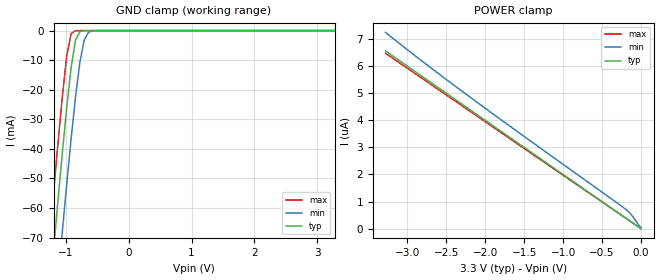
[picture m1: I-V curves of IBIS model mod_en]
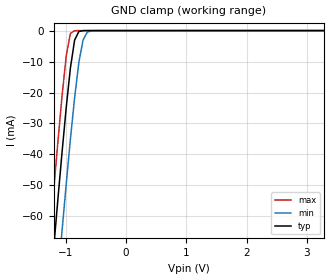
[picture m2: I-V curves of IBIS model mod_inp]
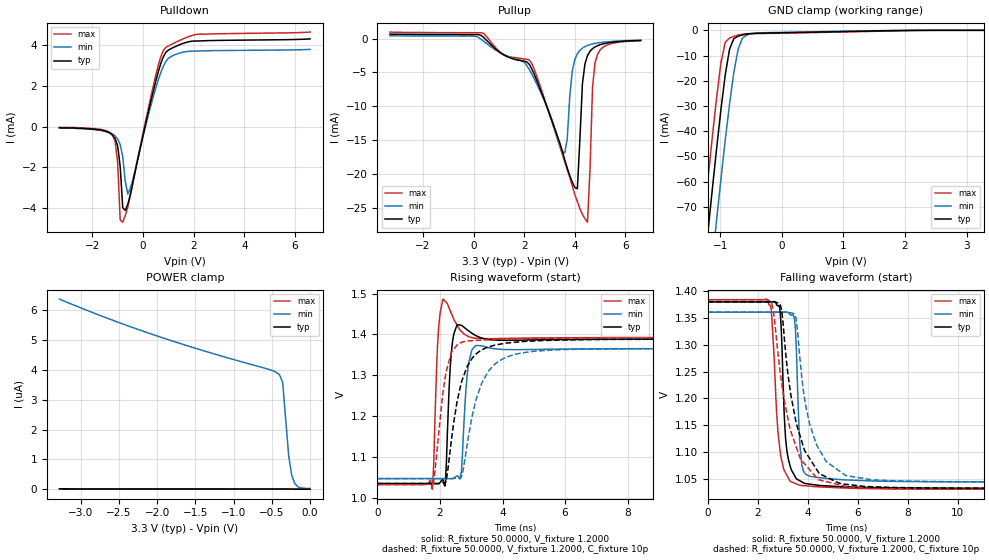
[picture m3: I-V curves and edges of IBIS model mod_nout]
| IBIS (I/O, Buffer, Information, Specification) Model, officially
| electronic behavioral standard for Buffer structures of digital pins.
[IBIS ver]  4.0
[File name] rhflvds2281.ibs
[File Rev]  1.0
[Date]   27 Jan 2015
[Source]   CAD & Design Services (Catania) - STMicroelectronics
[Notes]
   (Note1)  This IBIS model includes Ceramic Flat-64 package data
   (Note2)  This IBIS model has some Notes about the non-monotonicity
   of the I-V curves, but they are not indicative of problems
   inside the model;
[Copyright] (c) 2015 STMicroelectronics
|   Component RHFLVDS2281
[Component] RHFLVDS2281
[Manufacturer] STMicroelectronics
[Package]
| variable   typ   min   max
R_pkg   0.0   0.0   0.0
L_pkg   0.0H   0.0H   0.0H
C_pkg   0.0F   0.0F   0.0F
[Pin]  signal_name   model_name   R_pin   L_pin   C_pin
1   EN1   mod_en   NA   NA   NA
2   IN1P   mod_inp   NA   NA   NA
3   IN1N   mod_inn   NA   NA   NA
4   EN2   mod_en   NA   NA   NA
5   IN2P   mod_inp   NA   NA   NA
6   IN2N   mod_inn   NA   NA   NA
7   VCC   POWER   NA   NA   NA
8   GND   GND   NA   NA   NA
9   IN3P   mod_inp   NA   NA   NA
10   IN3N   mod_inn   NA   NA   NA
11   EN3   mod_en   NA   NA   NA
12   IN4P   mod_inp   NA   NA   NA
13   IN4N   mod_inn   NA   NA   NA
14   EN4   mod_en   NA   NA   NA
15   ENCK   mod_en   NA   NA   NA
16   CLKINP   mod_inp   NA   NA   NA
17   CLKINN   mod_inn   NA   NA   NA
18   GND   GND   NA   NA   NA
19   EN5   mod_en   NA   NA   NA
20   IN5P   mod_inp   NA   NA   NA
21   IN5N   mod_inn   NA   NA   NA
22   EN6   mod_en   NA   NA   NA
23   IN6P   mod_inp   NA   NA   NA
24   IN6N   mod_inn   NA   NA   NA
25   VCC   POWER   NA   NA   NA
26   GND   GND   NA   NA   NA
27   IN7P   mod_inp   NA   NA   NA
28   IN7N   mod_inn   NA   NA   NA
29   EN7   mod_en   NA   NA   NA
30   IN8P   mod_inp   NA   NA   NA
31   IN8N   mod_inn   NA   NA   NA
32   EN8   mod_en   NA   NA   NA
33   OUT8N   mod_nout   NA   NA   NA
34   OUT8P   mod_pout   NA   NA   NA
35   SL8   mod_sl   NA   NA   NA
36   OUT7N   mod_nout   NA   NA   NA
37   OUT7P   mod_pout   NA   NA   NA
38   SL7   mod_sl   NA   NA   NA
39   GND   GND   NA   NA   NA
40   VCC   POWER   NA   NA   NA
41   OUT6N   mod_nout   NA   NA   NA
42   OUT6P   mod_pout   NA   NA   NA
43   SL6   mod_sl   NA   NA   NA
44   OUT5N   mod_nout   NA   NA   NA
45   OUT5P   mod_pout   NA   NA   NA
46   SL5   mod_sl   NA   NA   NA
47   GND   GND   NA   NA   NA
48   CLKOUTN   mod_nout   NA   NA   NA
49   CLKOUTP   mod_pout   NA   NA   NA
50   VCC   POWER   NA   NA   NA
51   OUT4N   mod_nout   NA   NA   NA
52   OUT4P   mod_pout   NA   NA   NA
53   SL4   mod_sl   NA   NA   NA
54   OUT3N   mod_nout   NA   NA   NA
55   OUT3P   mod_pout   NA   NA   NA
56   SL3   mod_sl   NA   NA   NA
57   GND   GND   NA   NA   NA
58   VCC   POWER   NA   NA   NA
59   OUT2N   mod_nout   NA   NA   NA
60   OUT2P   mod_pout   NA   NA   NA
61   SL2   mod_sl   NA   NA   NA
62   OUT1N   mod_nout   NA   NA   NA
63   OUT1P   mod_pout   NA   NA   NA
64   SL1   mod_sl   NA   NA   NA
[Diff pin]  inv_pin   vdiff   tdelay_typ  tdelay_min  tdelay_max
2   3   200mV   0.0s   0.0s   0.0s
5   6   200mV   0.0s   0.0s   0.0s
9   10   200mV   0.0s   0.0s   0.0s
12   13   200mV   0.0s   0.0s   0.0s
16   17   200mV   0.0s   0.0s   0.0s
20   21   200mV   0.0s   0.0s   0.0s
23   24   200mV   0.0s   0.0s   0.0s
27   28   200mV   0.0s   0.0s   0.0s
30   31   200mV   0.0s   0.0s   0.0s
34   33   0.0V   0.0s   0.0s   0.0s
37   36   0.0V   0.0s   0.0s   0.0s
42   41   0.0V   0.0s   0.0s   0.0s
45   44   0.0V   0.0s   0.0s   0.0s
49   48   0.0V   0.0s   0.0s   0.0s
52   51   0.0V   0.0s   0.0s   0.0s
55   54   0.0V   0.0s   0.0s   0.0s
60   59   0.0V   0.0s   0.0s   0.0s
63   62   0.0V   0.0s   0.0s   0.0s
[Package Model]  302620_lvds2218
[Define Package Model]  302620_lvds2218
[Manufacturer]  STMicroelectronics
[OEM]  STMicroelectronics
[Description]  ceramic flat-64
[Number Of Pins]  64
[Pin Numbers]
|Pin Num   Terminal Name
1   | NET1:1
2   | NET2:2
3   | NET3:3
4   | NET4:4
5   | NET5:5
6   | NET6:6
7   | NET7:7
8   | NET8:8
9   | NET9:9
10   | NET10:10
11   | NET11:11
12   | NET12:12
13   | NET13:13
14   | NET14:14
15   | NET15:15
16   | NET16:16
17   | NET17:17
18   | NET18:18
19   | NET19:19
20   | NET20:20
21   | NET21:21
22   | NET22:22
23   | NET23:23
24   | NET24:24
25   | NET25:25
26   | NET26:26
27   | NET27:27
28   | NET28:28
29   | NET29:29
30   | NET30:30
31   | NET31:31
32   | NET32:32
33   | NET33:33
34   | NET34:34
35   | NET35:35
36   | NET36:36
37   | NET37:37
38   | NET38:38
39   | NET39:39
40   | NET40:40
41   | NET41:41
42   | NET42:42
43   | NET43:43
44   | NET44:44
45   | NET45:45
46   | NET46:46
47   | NET47:47
48   | NET48:48
49   | NET49:49
50   | NET50:50
51   | NET51:51
52   | NET52:52
53   | NET53:53
54   | NET54:54
55   | NET55:55
56   | NET56:56
57   | NET57:57
58   | NET58:58
59   | NET59:59
60   | NET60:60
61   | NET61:61
62   | NET62:62
63   | NET63:63
64   | NET64:64
[Model Data]
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[End Model Data]
[End Package Model]
| Models and submodels in the file (6): mod_en (Input), mod_inp (Input), mod_inn (Input), mod_nout (3-state), mod_pout (3-state), mod_sl (Input)
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|   Model mod_en
[Model]   mod_en
Model_type Input
Vinl   =   0.800V
Vinh   =   2.000V
C_comp   0.279pF   0.266pF   0.292pF
[Temperature Range]   25.0000   0.1250k   -55.0000
[Voltage Range]   3.3000V   3.0000V   3.6000V
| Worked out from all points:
|   GND clamp passes 1 mA (typ) near -0.80 V on its own axis
[GND_clamp]
|Voltage   I(typ)   I(min)   I(max)
-3.3V     -613.2mA   -637.8mA   -596mA
-1.27V    -91.5mA    -118.4mA   -72.02mA
-1.2V     -74.44mA   -101.4mA   -54.92mA
-1.13V    -57.71mA   -84.56mA   -38.25mA
-1.06V    -41.47mA   -68.06mA   -22.43mA
-990mV    -26.12mA   -52.01mA   -8.665mA
-920mV    -12.56mA   -36.67mA   -982.1uA
-850mV    -3.212mA   -22.55mA   -34.54uA
-780mV    -311.8uA   -10.71mA   -9.192uA
-710mV    -27.04uA   -3.134mA   -8.517uA
-570mV    -7.806uA   -73.26uA   -8.229uA
3.28V     -39.94nA   895.4nA    -631.5nA
[POWER_clamp]
|Voltage   I(typ)   I(min)   I(max)
-3.28V    6.559uA    7.243uA    6.473uA
-2.8V     5.599uA    6.161uA    5.526uA
-2.2V     4.4uA      4.867uA    4.342uA
-200mV    400.6nA    724.4nA    394.8nA
-120mV    240.6nA    502.7nA    236.9nA
0V        84.14pA    38.67nA    32.02pA
|   Model mod_inp
[Model]   mod_inp
Model_type Input
Vinl   =   1.100V
Vinh   =   1.300V
C_comp   2.433pF   1.683pF   2.667pF
[Temperature Range]   25.0000   0.1250k   -55.0000
[Voltage Range]   3.3000V   3.0000V   3.6000V
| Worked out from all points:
|   GND clamp passes 1 mA (typ) near -0.80 V on its own axis
[GND_clamp]
|Voltage   I(typ)   I(min)   I(max)
-3.3V     -582.8mA   -606.3mA   -566.5mA
-1.27V    -87.16mA   -112.8mA   -68.59mA
-1.2V     -70.94mA   -96.63mA   -52.32mA
-1.13V    -55.03mA   -80.64mA   -36.47mA
-1.06V    -39.58mA   -64.94mA   -21.4mA
-990mV    -24.95mA   -49.67mA   -8.241mA
-920mV    -12.01mA   -35.06mA   -889.7uA
-850mV    -3.049mA   -21.59mA   -24.72uA
-780mV    -287.4uA   -10.27mA   -2.037uA
-710mV    -19.39uA   -3.005mA   -1.412uA
-570mV    -1.205uA   -64.79uA   -1.125uA
3.28V     6.558uA    6.923uA    6.473uA
|   Model mod_nout
[Model]   mod_nout
Model_type 3-state
Polarity   Inverting
Enable   Active-Low
Vmeas  =   1.280V
Cref   =   10pF
C_comp   0.670pF   0.640pF   0.735pF
[Temperature Range]   25.0000   0.1250k   -55.0000
[Voltage Range]   3.3000V   3.0000V   3.6000V
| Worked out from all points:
|   slope of the pulldown table from 0 to 0.495 V, typ, clamps not added: 189 ohm
|   slope of the pullup table from 0 to 0.495 V, typ, clamps not added: 635 ohm
|   GND clamp passes 1 mA (typ) near -0.05 V on its own axis
|   rising waveform, R_fixture 50.0000, V_fixture 1.2000: 20-80 % time 112ps typ, 152ps min, 85.8ps max; typ from 1.03 V to 1.39 V
|   rising waveform, R_fixture 50.0000, V_fixture 1.2000, C_fixture 10p: 20-80 % time 540ps typ, 657ps min, 347ps max; typ from 1.03 V to 1.39 V
|   falling waveform, R_fixture 50.0000, V_fixture 1.2000: 20-80 % time 212ps typ, 160ps min, 287ps max; typ from 1.38 V to 1.03 V
|   falling waveform, R_fixture 50.0000, V_fixture 1.2000, C_fixture 10p: 20-80 % time 820ps typ, 782ps min, 856ps max; typ from 1.38 V to 1.03 V
[Pulldown]
|Voltage   I(typ)   I(min)   I(max)
-3.3V     -60uA      -70uA      -40uA
-1.2V     -426uA     -370uA     -431uA
-1.1V     -594uA     -462uA     -728uA
-1V       -953uA     -613uA     -1.784mA
-900mV    -1.969mA   -889uA     -4.592mA
-800mV    -3.985mA   -1.483mA   -4.695mA
-700mV    -4.113mA   -2.688mA   -4.37mA
-600mV    -3.813mA   -3.315mA   -3.95mA
500mV     2.207mA    1.874mA    2.487mA
900mV     3.636mA    3.189mA    3.875mA
2.2V      4.197mA    3.707mA    4.534mA
6.6V      4.298mA    3.785mA    4.633mA
[Pullup]
|Voltage   I(typ)   I(min)   I(max)
-3.3V     648.5uA    400.1uA    948.4uA
100mV     580uA      314.9uA    848.8uA
2.2V      -3.798mA   -4.575mA   -3.171mA
3.6V      -17.93mA   -16.93mA   -18.2mA
3.9V      -21.25mA   -4.76mA    -21.81mA
4.1V      -22.23mA   -2.252mA   -24.09mA
4.3V      -6.681mA   -1.42mA    -26mA
4.5V      -2.525mA   -1.04mA    -27.16mA
4.6V      -1.88mA    -910uA     -19.26mA
4.7V      -1.5mA     -810uA     -7.122mA
4.8V      -1.24mA    -720uA     -3.553mA
6.6V      -290uA     -260uA     -310uA
[GND_clamp]
|Voltage   I(typ)   I(min)   I(max)
-3.3V     -618mA     -644.4mA   -599.6mA
-1.27V    -96.79mA   -125.4mA   -76.01mA
-1.2V     -79.78mA   -108.4mA   -58.97mA
-1.06V    -46.87mA   -75.13mA   -26.67mA
-990mV    -31.49mA   -59.06mA   -12.94mA
-920mV    -17.71mA   -43.62mA   -4.778mA
-850mV    -7.485mA   -29.22mA   -3.049mA
-780mV    -3.3mA     -16.64mA   -2.381mA
-710mV    -2.307mA   -7.455mA   -1.88mA
-640mV    -1.824mA   -3.103mA   -1.539mA
-570mV    -1.491mA   -1.839mA   -1.352mA
3.28V     398.8pA    1.1uA      344.5pA
[POWER_clamp]
|Voltage   I(typ)   I(min)   I(max)
-3.28V    11.12nA    6.375uA    879.4pA
-2.68V    9.647nA    5.759uA    798.9pA
-2.04V    8.295nA    5.171uA    713.1pA
-560mV    5.839nA    4.032uA    514.6pA
-440mV    5.672nA    3.914uA    498.4pA
-400mV    5.615nA    3.831uA    492.8pA
-360mV    5.552nA    3.594uA    486.1pA
-280mV    5.327nA    1.1uA      469.9pA
-240mV    4.607nA    456.8nA    448.7pA
-200mV    1.988nA    184.6nA    409.6pA
-160mV    800.9pA    80.06nA    397.9pA
0V        401.5pA    24.41nA    379.3pA
[Ramp]
| variable   typ   min   max
dV/dt_r  0.2630/0.2424n   0.2113/0.3499n   0.3262/0.1812n
dV/dt_f  0.1093/71.0793p   0.1010/0.1209n   0.1112/69.1504p
R_load = 50.0000
[Rising Waveform]
R_fixture= 50.0000
V_fixture= 1.2000
V_fixture_min= 1.2000
V_fixture_max= 1.2000
|time   V(typ)   V(min)   V(max)
0s        1.035V     1.047V     1.033V
1.755ns   1.035V     1.047V     1.022V
1.92ns    1.035V     1.047V     1.37V
2.1ns     1.044V     1.047V     1.486V
2.175ns   1.04V      1.047V     1.48V
2.355ns   1.348V     1.047V     1.453V
2.55ns    1.424V     1.054V     1.422V
2.895ns   1.41V      1.316V     1.396V
3.135ns   1.398V     1.372V     1.391V
15ns      1.388V     1.365V     1.392V
[Rising Waveform]
R_fixture= 50.0000
V_fixture= 1.2000
V_fixture_min= 1.2000
V_fixture_max= 1.2000
C_fixture=10p
|time   V(typ)   V(min)   V(max)
0s        1.035V     1.047V     1.033V
1.755ns   1.035V     1.047V     1.032V
1.83ns    1.035V     1.047V     1.059V
2.19ns    1.039V     1.047V     1.306V
2.52ns    1.223V     1.049V     1.371V
2.73ns    1.293V     1.064V     1.382V
3.03ns    1.342V     1.2V       1.385V
3.33ns    1.362V     1.28V      1.386V
4.26ns    1.38V      1.348V     1.389V
15ns      1.388V     1.365V     1.392V
[Falling Waveform]
R_fixture= 50.0000
V_fixture= 1.2000
V_fixture_min= 1.2000
V_fixture_max= 1.2000
|time   V(typ)   V(min)   V(max)
0s        1.379V     1.36V      1.383V
2.505ns   1.379V     1.36V      1.373V
2.865ns   1.37V      1.36V      1.112V
2.94ns    1.321V     1.36V      1.087V
3.105ns   1.127V     1.361V     1.062V
3.315ns   1.07V      1.355V     1.046V
3.495ns   1.054V     1.332V     1.042V
3.675ns   1.047V     1.116V     1.039V
3.915ns   1.042V     1.059V     1.038V
15ns      1.033V     1.045V     1.032V
[Falling Waveform]
R_fixture= 50.0000
V_fixture= 1.2000
V_fixture_min= 1.2000
V_fixture_max= 1.2000
C_fixture=10p
|time   V(typ)   V(min)   V(max)
0s        1.379V     1.36V      1.383V
2.46ns    1.379V     1.36V      1.381V
2.64ns    1.379V     1.36V      1.355V
2.88ns    1.375V     1.36V      1.253V
3.51ns    1.16V      1.351V     1.113V
3.9ns     1.101V     1.19V      1.077V
4.41ns    1.064V     1.109V     1.049V
5.52ns    1.04V      1.057V     1.037V
6.57ns    1.036V     1.049V     1.033V
15ns      1.033V     1.045V     1.032V
